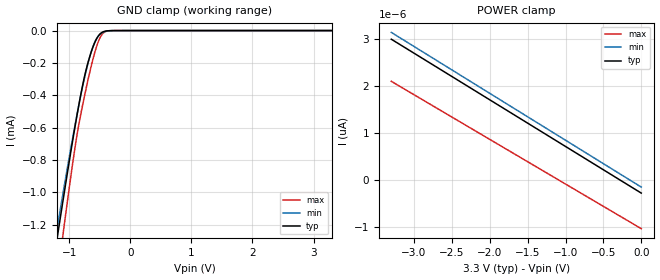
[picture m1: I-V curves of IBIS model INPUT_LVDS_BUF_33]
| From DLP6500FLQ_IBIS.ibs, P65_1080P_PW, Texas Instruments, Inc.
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[Model]   INPUT_LVDS_BUF_33
Model_type  Input
Vinl=0.70
Vinh=2.00
| variable   typ   min   max
C_comp   0.47pF   0.41pF   0.51pF
[Temperature Range]   40   140   -40
| Ambient temperature   25   125   -40
[Voltage range]   3.3   3   3.6
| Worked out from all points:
|   GND clamp passes 1 mA (typ) near -1.08 V on its own axis
[GND Clamp]
| INPUT_LVDS_BUF_33
|   Voltage   I(typ)   I(min)   I(max)
-3.3V     -6.735mA   -6.438mA   -8.022mA
-1.21V    -1.319mA   -1.257mA   -1.581mA
-1.18V    -1.246mA   -1.188mA   -1.493mA
-1.12V    -1.1mA     -1.052mA   -1.319mA
-1.075V   -991.9uA   -951.1uA   -1.19mA
-885mV    -554.6uA   -547.4uA   -678.8uA
-740mV    -271.3uA   -278.7uA   -390.1uA
-595mV    -87.5uA    -84.44uA   -155.8uA
-520mV    -32.39uA   -33.33uA   -66.3uA
-450mV    -8.917uA   -11.77uA   -18.58uA
-265mV    -94.77nA   -339.3nA   -72.12nA
3.3V      293.4pA    15.6nA     68.11pA
[POWER Clamp]
| INPUT_LVDS_BUF_33
|   Voltage   I(typ)   I(min)   I(max)
-3.3V     3.003pA    3.148pA    2.105pA
-2.405V   2.113pA    2.254pA    1.252pA
-1.685V   1.397pA    1.534pA    566.5fA
-48.03fV  -278.9fA   -151.1fA   -1.037pA
